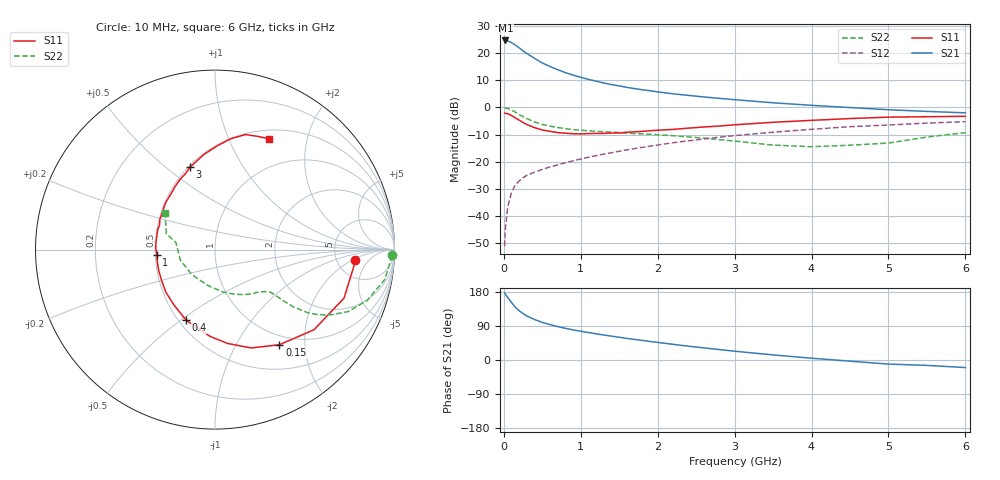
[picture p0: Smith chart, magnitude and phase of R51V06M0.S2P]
! SIEMENS Small Signal Semiconductors
! BFR183
! Si NPN RF Bipolar Junction Transistor in SOT23
! VCE = 1 V  IC = 6 mA
! Common Emitter S-Parameters:  May  1996
# GHz  S  MA  R  50
!  f  S11  S21  S12  S22
! GHz  MAG  ANG  MAG  ANG  MAG  ANG  MAG  ANG
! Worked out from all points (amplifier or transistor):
!   36 points, 10 MHz to 6 GHz, reference 50 ohm
!   highest |S21| = 24.6 dB at 20 MHz (marker M1)
!   |S21| within 3 dB of that: start of sweep to 212.8 MHz
!   unconditionally stable (mu >= 1): 886 MHz to 2.855 GHz
!   at 250 MHz: K = 0.48, MSG = 23.3 dB, |S12| = -25.8 dB
!   at 1.4 GHz: K = 1.08, MAG = 10.8 dB, |S12| = -16.7 dB
!   at 6 GHz: K = 0.93, MSG = 1.6 dB, |S12| = -5.2 dB
!   S11 on the Smith chart (normalised r, x): 10 MHz: 7.57, -2.32; 150 MHz: 0.85, -1.53; 400 MHz: 0.55, -0.52; 1 GHz: 0.51, -0.03; 3 GHz: 0.51, +0.61; 6 GHz: 0.61, +1.42
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0.01  0.7848 -4.3  16.95 177.2  0.0028 92.4  0.9848 -1.9
0.02  0.7761 -8.2  17.08 173.8  0.0059 85.8  0.9787 -4.0
0.05  0.7681 -20.6  16.86 164.9  0.0148 79.8  0.9603 -10.0
0.1  0.7097 -39.0  15.52 151.6  0.0273 71.6  0.8938 -18.5
0.15  0.64 -55.9  14.04 139.1  0.0373 64.9  0.8175 -25.0
0.2  0.5835 -69.9  12.49 129.9  0.0448 60.9  0.7403 -29.4
0.25  0.5278 -82.3  10.99 122.4  0.051 57.4  0.6762 -32.4
0.3  0.4849 -93.1  9.806 116.0  0.0564 56.4  0.6228 -34.3
0.4  0.4245 -112.4  7.986 106.8  0.0646 54.7  0.5397 -36.2
0.5  0.385 -126.1  6.583 99.3  0.0721 54.8  0.4857 -36.7
0.6  0.363 -138.7  5.65 93.4  0.0804 54.9  0.453 -36.9
0.8  0.335 -159.3  4.375 83.6  0.0959 56.1  0.4063 -37.3
1  0.3254 -175.1  3.576 75.9  0.1127 57.2  0.3808 -38.1
1.1  0.3306 178.0  3.285 72.5  0.1212 57.5  0.3717 -39.2
1.3  0.3333 166.1  2.816 66.0  0.1388 57.3  0.3571 -41.0
1.6  0.3505 151.2  2.341 56.9  0.1658 56.6  0.3371 -45.1
2.2  0.3944 128.7  1.782 41.4  0.2239 53.1  0.3021 -56.1
3  0.4791 107.0  1.389 23.2  0.3033 45.0  0.2407 -79.4
3.5  0.533 96.8  1.218 13.4  0.3499 38.8  0.2026 -102.5
4.5  0.6242 81.9  0.995 -3.1  0.4424 26.1  0.2016 -162.9
5.5  0.6749 69.1  0.845 -14.2  0.5151 14.0  0.2856 161.9
6  0.6869 63.9  0.795 -20.0  0.5476 6.2  0.3437 143.9
